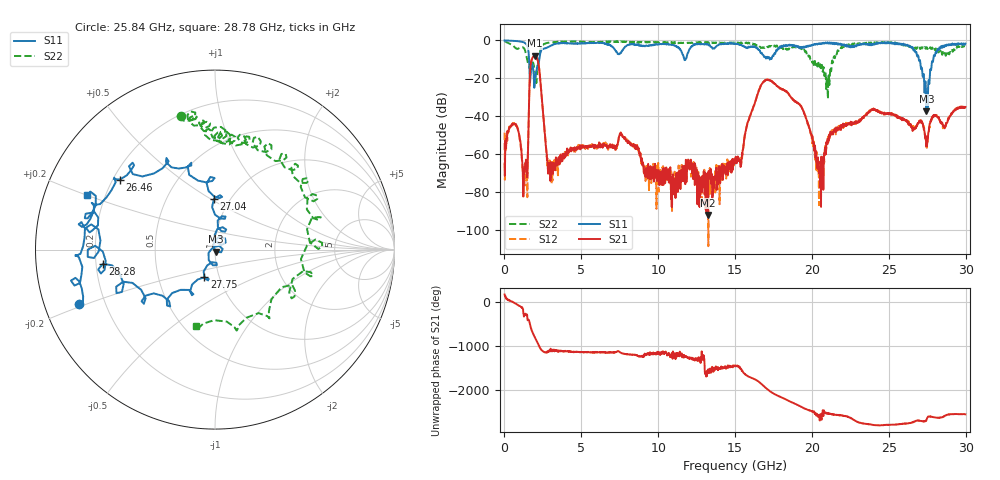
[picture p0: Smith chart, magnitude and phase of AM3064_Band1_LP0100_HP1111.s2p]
# Hz S DB R 50.0
!freq dBS11 angS11 dBS21 angS21 dBS12 angS12 dBS22 angS22
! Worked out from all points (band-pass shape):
!   1600 points, 10 MHz to 29.98 GHz, reference 50 ohm
!   highest |S21| = -8.09 dB at 1.978 GHz (marker M1); lowest = -91.9 dB at 13.24 GHz (marker M2)
!   |S21| within 3 dB of the highest: 1.742 GHz to 2.183 GHz (441 MHz wide, 22.5 % of centre)
!   lowest |S11| = -37.3 dB at 27.45 GHz (marker M3), VSWR 1.03, Z = 50.7 - j1.2 ohm
!   |S11| at or under -10 dB: 1.6 GHz to 2.267 GHz (667.4 MHz wide, 34.5 % of centre); 11.7 GHz to 11.78 GHz (79.62 MHz wide, 0.678 % of centre); 26.95 GHz to 27.89 GHz (939.7 MHz wide, 3.43 % of centre)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
!   |S22| runs from -30.8 to -0.4 dB; largest |S21 - S12| = 0.0092
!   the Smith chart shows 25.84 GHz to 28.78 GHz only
!   S11 on the Smith chart (normalised r, x): 25.84 GHz: 0.10, -0.19; 26.46 GHz: 0.23, +0.31; 27.04 GHz: 0.84, +0.52; 27.75 GHz: 0.85, -0.27; 28.28 GHz: 0.23, -0.06; 28.78 GHz: 0.13, +0.20
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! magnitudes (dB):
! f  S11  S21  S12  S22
! 10 MHz  0.0  -64.8  -48.6  -0.4
! 666 MHz  -0.3  -43.9  -43.5  -3.6
! 1.36 GHz  -1.5  -65.6  -67.3  -5.9
! 1.734 GHz  -15.3  -11.3  -11.2  -14.1
! 1.978 GHz  -21.4  -8.1  -8.1  -16.3
! 2.953 GHz  -3.1  -70.1  -63.2  -1.2
! 5.015 GHz  -1.5  -55.8  -56.3  -0.6
! 10 GHz  -2.0  -68.2  -64.5  -0.9
! 13.24 GHz  -2.1  -91.9  -78.4  -1.0
! 15 GHz  -1.9  -63.3  -65.2  -1.4
! 17.03 GHz  -9.3  -20.7  -20.8  -4.0
! 19.99 GHz  -2.7  -51.1  -51.6  -10.9
! 20.55 GHz  -1.7  -72.7  -75.9  -13.4
! 25 GHz  -1.0  -39.0  -38.3  -1.2
! 25.84 GHz  -1.8  -41.4  -41.8  -2.3
! 26.46 GHz  -3.6  -45.5  -45.2  -3.5
! 27.04 GHz  -10.9  -42.0  -42.7  -4.6
! 27.45 GHz  -37.3  -54.4  -56.1  -3.6
! 27.75 GHz  -15.6  -41.8  -41.5  -4.5
! 28.28 GHz  -4.0  -41.6  -41.3  -5.2
! 28.78 GHz  -2.2  -43.2  -42.9  -7.1
! 29.98 GHz  -1.6  -35.0  -35.0  -2.9
